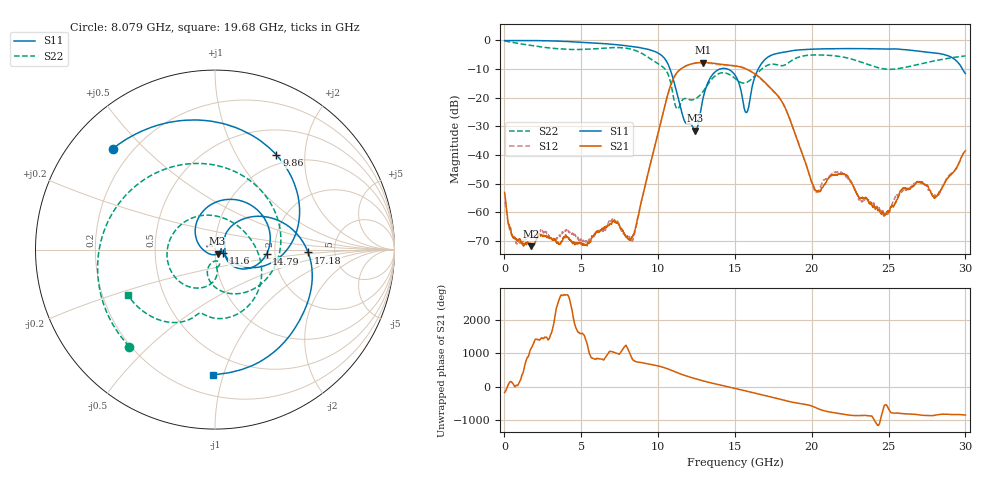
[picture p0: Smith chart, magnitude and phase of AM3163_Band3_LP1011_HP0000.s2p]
!Agilent Technologies,E8364B,MY43040894,A.07.50.67
!Agilent E8364B: A.07.50.67
!Date: Thursday, August 20, 2020 12:12:22
!Correction: S11(Full 2 Port(1,2))
!S21(Full 2 Port(1,2))
!S12(Full 2 Port(1,2))
!S22(Full 2 Port(1,2))
!S2P File: Measurements: S11, S21, S12, S22:
# Hz S  dB  R 50
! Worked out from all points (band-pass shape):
!   3201 points, 10 MHz to 30 GHz, reference 50 ohm
!   highest |S21| = -7.71 dB at 12.92 GHz (marker M1); lowest = -71.8 dB at 1.734 GHz (marker M2)
!   |S21| within 3 dB of the highest: 11.32 GHz to 16 GHz (4.684 GHz wide, 34.3 % of centre)
!   lowest |S11| = -31.4 dB at 12.42 GHz (marker M3), VSWR 1.06, Z = 51.4 - j2.33 ohm
!   |S11| at or under -10 dB: 10.78 GHz to 14.01 GHz (3.23 GHz wide, 26.1 % of centre); 14.53 GHz to 16.52 GHz (1.982 GHz wide, 12.8 % of centre); 29.81 GHz to end of sweep
!   |S22| runs from -24.0 to -0.2 dB; largest |S21 - S12| = 0.013
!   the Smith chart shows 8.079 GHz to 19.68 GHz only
!   S11 on the Smith chart (normalised r, x): 8.079 GHz: 0.13, +0.41; 9.86 GHz: 0.85, +1.48; 11.6 GHz: 1.09, -0.04; 14.79 GHz: 1.80, -0.10; 17.18 GHz: 3.15, -0.14; 19.68 GHz: 0.34, -0.92
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1e7  -0.04 -2.0  -53.06 -170.5  -56.28 163.0  -0.20 -5.4
1.734425e9  -0.03 -47.6  -71.84 58.0  -67.90 73.1  -1.77 -121.6
3.065231e9  -0.16 -83.8  -69.36 171.4  -69.23 57.6  -2.70 163.6
5.014581e9  -0.61 -135.6  -70.74 151.1  -70.23 30.8  -3.15 60.5
6.45785e9  -1.10 -174.9  -65.90 78.1  -66.34 101.3  -2.69 -22.5
8.079184e9  -1.93 135.3  -69.35 1.3  -68.69 137.4  -2.84 -131.5
9.859841e9  -4.03 57.0  -35.36 -84.6  -35.42 -85.0  -7.66 49.0
1.000979e10  -4.43 47.5  -32.10 -100.2  -32.16 -100.9  -8.16 28.0
1.160301e10  -26.29 -24.5  -9.51 -1.0  -9.54 -1.0  -20.67 -76.3
1.241836e10  -31.45 -57.7  -7.91 -118.7  -7.94 -118.7  -20.41 -86.4
1.291507e10  -20.44 162.3  -7.71 178.3  -7.75 178.0  -17.91 -84.2
1.373042e10  -10.87 77.3  -8.06 85.0  -8.31 85.2  -12.27 -118.8
1.478945e10  -10.81 -4.9  -8.75 -25.3  -8.72 -23.5  -12.38 149.2
1.5005e10  -12.09 -20.0  -8.90 -48.0  -8.78 -46.4  -13.25 125.9
1.575475e10  -25.16 8.4  -10.03 -129.6  -9.95 -129.9  -14.68 42.4
1.717928e10  -5.70 -1.8  -15.86 74.4  -16.00 75.6  -8.54 -65.9
1.968157e10  -3.13 -91.0  -44.19 -173.9  -43.96 -171.7  -5.22 -152.5
2.000958e10  -3.05 -99.7  -49.59 144.2  -49.74 146.2  -5.08 -164.7
2.25025e10  -2.84 -157.5  -49.00 -129.3  -48.98 -130.2  -6.37 100.3
2.500479e10  -3.00 144.4  -59.62 56.6  -60.18 161.8  -10.10 -38.2
2.73665e10  -3.95 78.8  -50.27 -134.0  -50.43 -128.9  -7.85 -159.1
3e10  -11.53 -28.1  -38.54 -121.8  -38.64 -121.7  -5.40 111.1
